FUNCTION_BLOCK IDENTControl_MF
VAR_INPUT
	pADR_IN:								PVOID;					(* Pointer array input data *)
	cbSIZE_IN:								UDINT;					(* Size array input data *)
	pADR_OUT:								PVOID;					(* Pointer array output data *)
	cbSIZE_OUT:								UDINT;					(* Size array output data *)
    I_T_Timeout 							: TIME := T#10S;   		// Timeout to check command responses
    I_b_StartRead 							: BOOL;   				// Trigger to start read command
    I_b_StartWrite 							: BOOL;   				// Trigger to start write command
    I_b_StartSpecialCommand 				: BOOL;   				// Trigger to start special command (user defined command)
    I_b_UserMemory_UID 						: BOOL;   				//0 := access to User Memory; 1 := access to UID/Fixcode
    I_b_EPC									: BOOL;					//0 := configuration done by Head1UserMemoryUID active; 1 := access to UII/EPC Code (UHF only)
	I_b_SingleEnhanced 						: BOOL;   				// 0 = Single command (one-time) ; 1 = Enhanced command (permanent)
    I_b_Quit 								: BOOL;   				// Trigger to start Quit command (abort Enhanced command)
    I_w_StartAddress 						: WORD;   				// Startaddress of memory access 
    I_i_WordNumber 							: INT;   				// Number of blocks
    I_w_TagType 							: WORD;    				// TagType
END_VAR
VAR_OUTPUT
	O_b_Done 								: BOOL;   				//0 = tag leave detection zone (Enhanced); 1 = tag access successfully executed
    O_b_NoDataCarrier 						: BOOL;   				//0 = tag inside/enter detection zone; 1 = no tag or tag leave detection zone
    O_b_Busy 								: BOOL;   				//0 = no command actiive; 1 = command active
    O_b_Finish 								: BOOL;   				//0 = command active; 1 = command finished
    O_b_Error 								: BOOL;   				//0 = no error state; 1 = error state active; check status value
    O_B_Status 								: BYTE;   				//Status value of the command response; error information
	O_B_ReplyCounter 						: BYTE;					//Counter of the command responses; increment each new response
END_VAR
   VAR_IN_OUT 
    IO_b_SetRestart 						: BOOL;   				//Trigger initialisation routine
    IO_b_InitFinish 						: BOOL;   				//Initialisation routine finished
	IO_b_NewData							: BOOL;  	
	UserData 								: IDENTControl_UserData_IUH_MF;//Data block for read/write data
 	END_VAR
VAR
	INDATA 									: ARRAY[0..253] OF BYTE;
	OUTDATA 								: ARRAY[0..253] OF BYTE;
	UpdateSlave_IN							: BOOL;
    MASK_UPDATEBIT_SLAVE 					: BYTE := 1;
    MASK_UPDATEBIT_MASTER 					: BYTE := 2;
    MASK_DELETEBIT 							: BYTE := 4;
	
	statEdgeA								: BOOL;
	statEdgeB								: BOOL;
	statFlagC								: BOOL;
	
	Counter_FP								: INT;
	
	Head_ExistTC							: BOOL;
	Head_NotExist							: BOOL;
	Head_Done								: BOOL;
	Head_Error								: BOOL;
	Head_Busy								: BOOL;
	Head_SglCmdActive						: BOOL;
	Head_EnhCmdActive						: BOOL;
	Head_QuitCmdActive						: BOOL;
	Head_ReadCmdActive						: BOOL;
	Head_SpecialCmdActive					: BOOL;
	Head_NewData							: BOOL;
	Head_TimeoutActive						: BOOL;
	Head_TimeoutOccurred					: BOOL;
	Head_TransfToHead						: BOOL;
	Head_SendOK								: BOOL;
	Head_Execute							: BOOL;
	Head_Receive_OK							: BOOL;
	Head_WriteCmdActive						: BOOL;
	
	RTRIG_Read:									R_TRIG;					(* function block detects positive edge Read Command *)
	RTRIG_Write: 								R_TRIG;					(* function block detects positive edge Write Command *)
	RTRIG_Quit : 								R_TRIG;					(* function block detects positive edge Quit Command *)
	RTRIG_SpecialCommand: 						R_TRIG;					(* function block detects positive edge Special Command *)
	RTRIG_SetRestart: 							R_TRIG;					(* function block detects positive edge SetRestart *)
	
	STATE_INIT 								: USINT;
    STATE_CMD 								: USINT;
	
	Watchdog:									TON;
	i										: INT := 0;
	FragmentCounter_1						: INT;
	StartReadDataTransmission				: Bool;
	SingleCommandFinished					: BOOL;
	NumberTags								: DWORD;
END_VAR

	(*
	#############################################################################################
	
	General Header
	------------------------------------------------------------------------------------------
	Short description:  Function Block for IC-KP2-2HB21-2V1D EtherCAT with MultiFrame Protocol
	Version:            3.0
	Name:               Function block for IC-KP2-2HB21-2V1D EtherCAT with MultiFrame Protocol
	Date:               2024-09-19
	Company:            Pepperl+Fuchs SE
	Author:             Karsten Reinhardt
	EMail:              kreinhardt@de.pepperl-fuchs.com
	Phone:              +49 (0) 621 776 1736
	
		Changes 3.0: first release
	    - based on the SingleFrame version with adoption to MultiFrame
		- contains further commands which not supported by the UHF system
		- reading and writing is done with the 16 Bit commands
	
	
	*)


(*Read in process data; copy into #INDATA structure*)
MEMCPY(ADR(INDATA), pADR_IN, cbSIZE_IN); (* Receive complete Input-Telegram from IdentControl *)

(* Check every cycle if a new telegram is available *)
	IF (((INDATA[0]) AND MASK_UPDATEBIT_SLAVE) = ((OUTDATA[0] AND MASK_UPDATEBIT_SLAVE))) THEN
	    Head_Receive_OK                                 := TRUE;    (* inform PLC, that a new telegram is available *)
	    
	ELSE
	    Head_Receive_OK                                 := FALSE;   (* inform PLC, that no new telegram is available *)
	END_IF;
	(*Copy Update slave bit into internal variable*)
	UpdateSlave_IN 										:= InData[0].0;
	(*Trigger for positive edge on Update slave bit*)
	statEdgeA 											:= UpdateSlave_IN AND NOT statFlagC;
	(*Trigger for negative edge on Update slave bit*)
	statEdgeB 											:= NOT UpdateSlave_IN AND statFlagC;
	
	statFlagC 											:= UpdateSlave_IN;
	
	//generate Testcounter
	IF (statEdgeA = TRUE) OR (statEdgeB = TRUE) THEN
	    Counter_FP 										:= Counter_FP + 1;     // increment each new response telegram
	END_IF;

	//--------------------------------------------
	
	       O_B_Status 							:= INDATA[4];
			O_B_ReplyCounter 					:= INDATA[5];	
	
		//first response telegram after send command
	    IF Counter_FP = 1 THEN
	        FragmentCounter_1 							:= 16#0;                  //Fragment counter of first response telegram                    
	        IF ((INDATA[4] = 16#00) OR (INDATA[4] = 16#04)) AND (INDATA[2] <> 16#02) THEN              //Status
	        FOR i:=0 TO 245 BY 1 DO
			UserData.ReadData[i]						:= INDATA[i+8];
			END_FOR;
				StartReadDataTransmission 				:= TRUE;
	        END_IF;
	        
	        IF FragmentCounter_1 >= 16#00 AND INDATA[4] = 16#00 THEN
	            O_b_NoDataCarrier 						:= FALSE;
	            O_b_Error 								:= FALSE;
	        END_IF;
	        
	        IF FragmentCounter_1 = 16#00 THEN
	            IF INDATA[4] = 16#05 THEN  // No Tag
	                HEAD_Done 							:= FALSE;
	                HEAD_NewData 						:= TRUE;
	                HEAD_Execute 						:= FALSE;
	                HEAD_TimeoutActive 					:= FALSE;
	                O_b_NoDataCarrier 					:= TRUE;
	                Counter_FP 							:= 16#00;
	             	//   O_B_Status 							:= INDATA[4];
					//	O_B_ReplyCounter 					:= INDATA[5];
	                O_b_Done 							:= FALSE;
	                O_b_Error 							:= FALSE;
					FOR i:=0 TO 55 BY 1 DO
					UserData.EPC_LeaveTag[i]			:= INDATA[i+8];
					END_FOR;
					IO_b_NewData 						:= TRUE;
	              //  IF #statEdge1 = True THEN
	            END_IF;
	            IF  INDATA[4] = 16#00 THEN
	                HEAD_Done 							:= FALSE;
	                HEAD_NewData 						:= TRUE;
	                HEAD_Execute 						:= FALSE;
	                HEAD_TimeoutActive 					:= FALSE;
	                O_b_NoDataCarrier 					:= FALSE;
	             //   O_B_Status 							:= INDATA[4];
				//	O_B_ReplyCounter 					:= INDATA[5];
	                O_b_Done 							:= TRUE;
	                O_b_Error 							:= FALSE;
					IO_b_NewData 						:= TRUE;
	              //  IF #statEdge1 = True AND #Resp_Telegram_1[5] <> 16#04 AND #Resp_Telegram_1[6] = 16#00  AND NOT #HEAD.QuitCmdActive = True THEN
	            END_IF;
	            IF  INDATA[4] = 16#0B THEN
					FOR i:=0 TO 4 BY 1 DO
					UserData.TagInformation[i]				:= INDATA[i+8];
					END_FOR;
					IO_b_NewData 						:= TRUE;
	            END_IF;
				IF HEAD_SglCmdActive = TRUE AND INDATA[4] = 16#0F  THEN
	                O_b_Finish 							:= TRUE;
	                O_b_Done 							:= TRUE;
	                O_b_Busy 							:= FALSE;
	                HEAD_SglCmdActive 					:= FALSE;
	                HEAD_ReadCmdActive 					:= FALSE;
					HEAD_WriteCmdActive 					:= FALSE;
					HEAD_TimeoutActive 					:= FALSE;
					HEAD_Busy 							:= FALSE;
					HEAD_Execute 						:= FALSE;
					FOR i:=0 TO 3 BY 1 DO
					UserData.NumberTags[i]				:= INDATA[i+8];
					END_FOR;
					NumberTags							:= SHL (BYTE_TO_DWORD(UserData.NumberTags[0]), 24) OR 
														SHL (BYTE_TO_DWORD(UserData.NumberTags[1]), 16) OR 
														SHL (BYTE_TO_DWORD(UserData.NumberTags[2]), 8) OR 
														BYTE_TO_DWORD(UserData.NumberTags[3]);
					IF Numbertags = 16#30303030 THEN
					O_b_NoDataCarrier 					:= TRUE;
	                Counter_FP 							:= 16#00;
	            //    O_B_Status 							:= INDATA[4];
				//	O_B_ReplyCounter 					:= INDATA[5];
	                O_b_Error 							:= FALSE;	
					END_IF;		
					IO_b_NewData 						:= TRUE;						
	            END_IF;
				IF HEAD_SglCmdActive = TRUE AND INDATA[4] = 16#04 THEN
	                O_b_Finish 							:= TRUE;
	                O_b_Done 							:= TRUE;
	                O_b_Busy 							:= FALSE;
	                HEAD_SglCmdActive 					:= FALSE;
	                HEAD_ReadCmdActive 					:= FALSE;
	                HEAD_TimeoutActive 					:= FALSE;
	                HEAD_Execute 						:= FALSE;
	                HEAD_Busy 							:= FALSE;
	                O_b_Error 							:= TRUE;
	            //    O_B_Status 							:= INDATA[4];
				//	O_B_ReplyCounter 					:= INDATA[5];
	           		IO_b_NewData 						:= TRUE;
				END_IF;
	            IF HEAD_EnhCmdActive = TRUE AND INDATA[4] = 16#04 THEN
	                O_b_Done 							:= TRUE;
	                HEAD_ReadCmdActive 					:= FALSE;
	                HEAD_TimeoutActive 					:= FALSE;
	                O_b_Error 							:= TRUE;
	             //   O_B_Status 							:= INDATA[4];
				//	O_B_ReplyCounter 					:= INDATA[5];
	                Counter_FP 							:= 16#00;
					IO_b_NewData 						:= TRUE;
	            END_IF;
				IF HEAD_WriteCmdActive = TRUE AND INDATA[4] = 16#00 THEN
					FOR i:=0 TO 55 BY 1 DO
					UserData.EPC_WrittenTag[i]			:= INDATA[i+8];
					END_FOR;
				END_IF;
				IF INDATA[4] = 16#04 THEN
					O_b_Error 							:= TRUE;
				//	O_B_Status 							:= INDATA[4];
				//	O_B_ReplyCounter 					:= INDATA[5];
				END_IF
	        END_IF;
	    END_IF;
		Counter_FP 										:= 16#00;
	
	//-------------------------------------------	
		
	
	(* PLC always copy the inverted Update Slave bit from INPUT to OUTPUT *)
	(*  is now allowed to send a new telegram *)
	OUTDATA[0]                                         	:= ((OutData[0] AND (NOT MASK_UPDATEBIT_SLAVE)) OR ((NOT InData[0]) AND MASK_UPDATEBIT_SLAVE));
	
	(* Define Trigger inputs as rising edges *)        
	RTRIG_SetRestart(CLK                               	:=  IO_b_SetRestart);      (*SetRestart Input*)
	RTRIG_Quit(CLK                                     	:=  I_b_Quit);             (*Quit Input*)
	RTRIG_Read(CLK                                     	:=  I_b_StartRead);        (*Read Input*)
	RTRIG_Write(CLK                                    	:=  I_b_StartWrite);       (*Write Input*)
	RTRIG_SpecialCommand(CLK                           	:=  I_b_StartSpecialCommand);   (*SpecialCommand Input*)
	
	
	(* Handling of the SetRestart Routine
	- routine consist of the flip of the Delete Bit and the execution of the Change Tag command
	*) 
	IF RTRIG_SetRestart.Q THEN                                                     (*Check positive edge on SetRestart input*)
	    STATE_INIT                                     	:= 1;
	    STATE_CMD                                      	:= 0;
	    Counter_FP                                     	:= 0;
	END_IF;
	
	CASE STATE_INIT OF
	        
	    0:  (* ********************** Idle state ******************* *)
	        ;
	    1:  (* ********************** Initialize variables  ******************* *)
	        
	        (*Reset internal variables and Outputs*) 
	        IO_b_InitFinish                            	:= FALSE;
	        HEAD_ExistTC                               	:= FALSE;
	        HEAD_NotExist                              	:= FALSE;
	        HEAD_Done                                  	:= FALSE;
	        O_b_Done                                   	:= FALSE;
	        HEAD_Error                                 	:= FALSE;
	        O_b_Error                                  	:= FALSE;
	        HEAD_Busy                                  	:= FALSE;
	        O_b_Busy                                   	:= FALSE;
	        HEAD_SglCmdActive                          	:= FALSE;
	        HEAD_EnhCmdActive                          	:= FALSE;
	        HEAD_QuitCmdActive                         	:= FALSE;
	        HEAD_ReadCmdActive                         	:= FALSE;
	        HEAD_SpecialCmdActive                      	:= FALSE;
	        HEAD_NewData                               	:= FALSE;
	        HEAD_TimeoutActive                         	:= FALSE;
	        HEAD_TimeoutOccurred                       	:= FALSE;
	        HEAD_TransfToHead                          	:= FALSE;
	        HEAD_SendOK                                	:= FALSE;
	        HEAD_Execute                               	:= FALSE;
	        HEAD_Receive_OK                            	:= FALSE;
	        HEAD_WriteCmdActive                        	:= FALSE;
	        O_b_NoDataCarrier                          	:= FALSE;
	        O_b_Finish                                 	:= FALSE;
			IO_b_NewData 									:= FALSE;
			
			FOR i:=0 TO 245 BY 1 DO
		    UserData.WriteData[i]                       := 16#00;
			END_FOR;
			FOR i:=0 TO 245 BY 1 DO
		    UserData.ReadData[i]                       := 16#00;
			END_FOR;
	        FOR i:=0 TO 3 BY 1 DO
		    UserData.NumberTags[i]                       := 16#00;
			END_FOR;
			FOR i:=0 TO 4 BY 1 DO
		    UserData.TagInformation[i]                       := 16#00;
			END_FOR;
			FOR i:=0 TO 55 BY 1 DO
		    UserData.EPC_WrittenTag[i]                       := 16#00;
			END_FOR;
			FOR i:=0 TO 55 BY 1 DO
		    UserData.EPC_LeaveTag[i]                       := 16#00;
			END_FOR;
	       
	        STATE_INIT                                 	:= STATE_INIT + 1;                 (* Go to next state *)
	        
	        Counter_FP := 0;
	
	        
	    2: (* ****************** Delete internal FIFO Memory / telegrams of IC-KP2-2HB21 *************** *)
	        
	        (* Set Deletebit *)
	        OutData[0]                                 	:= ((OutData[0] AND (NOT MASK_DELETEBIT)) OR ((NOT OutData[0]) AND MASK_DELETEBIT));    (* Delete old telegrams in identsystem *)
	        
	        STATE_INIT                                 	:= STATE_INIT + 1;                 (* Go to next state *)
	        
	    3: (* ******************** Wait for delete bit in INPUTS equals OUTPUTS **************** *)
	        
	        IF ((OutData[0] AND MASK_DELETEBIT) = (( InData[0] AND MASK_DELETEBIT))) THEN       (*Check if the value of the Delete Bit is identically in input and output*)
	            STATE_INIT                             	:= STATE_INIT + 1;                 (* Go to next state *)
	        END_IF;
	        
	    4: (* ***************** Send Change Tag Command; stop command execution *************** *)
	        
	        (* Configure Change Tag command in OutData structure *)
	        OutData[1]                                 	:= 16#00;           (*unused*)
	        OutData[2]                                 	:= 16#04;           (*CommandCode CT*)
	        OutData[3]                                 	:= 16#00;           (*unused*)
	        OutData[4]                                 	:= WORD_TO_BYTE(SHR(I_w_TagType,8));           (*TagType High Byte*)
	        OutData[5]                                 	:= WORD_TO_BYTE(I_w_TagType);           (*TagType Low Byte*)
			FOR i:=6 TO 253 BY 1 DO
		    OutData[i]                                 	:= 16#00;
			END_FOR;	        	        
	        HEAD_Busy                                  	:= TRUE;
	        O_b_Busy                                   	:= TRUE;
	        HEAD_Done                                  	:= FALSE;
	        O_b_Done                                   	:= FALSE;
	        HEAD_TimeoutActive                         	:= TRUE;
	        HEAD_SglCmdActive                          	:= TRUE;
	        HEAD_EnhCmdActive                          	:= FALSE;
	        HEAD_Execute                               	:= TRUE;
	        HEAD_TransfToHead                          	:= TRUE;
	        
	        (* Handling of Handshake process for sending a new command *)
	        (* Check if IC-KP2-2HB21 is able to receive a new telegram; 
	        IC-KP2-2HB21 is able to receive new telegrams if the value of the UpdateBit_Master of the Input and Output is different *)
	        IF ((OutData[0] AND MASK_UPDATEBIT_MASTER) <> (InData[0] AND MASK_UPDATEBIT_MASTER)) THEN  (* Receiver (IC-KP2-2HB21) accepts a new Telegram *)
	                        (* Invert Updatebit master in order to signalize a new telegram is available *)
	            OutData[0]                             	:= (OutData[0] AND (NOT MASK_UPDATEBIT_MASTER)) OR (InData[0] AND MASK_UPDATEBIT_MASTER);
	            HEAD_SendOK                            	:= TRUE;
	        ELSE
	            HEAD_SendOK                            	:= FALSE;  (* Receiver (IC-KP2-2HB21) doesnt't accept a new Telegram *)
	        END_IF;
	        
	        (* Send OutData field with Quit command to IC-KP2-2HB21 *)
	        IF HEAD_SendOK THEN
	            
	            HEAD_TransfToHead                      	:= FALSE;
	            STATE_INIT                             	:= STATE_INIT + 1; (* Go to next state *)
	        END_IF;
	        
	    5: (* ******************** Wait for Quit command response ************************ *)
	        IF HEAD_Receive_OK THEN (*If new telegram from IC-KP2-2HB21 is available*)
	            
	            HEAD_NewData                           	:= TRUE;
	           // O_B_Status                             	:= InData[4];          (*Copy received status value to Output variable Status*)
	           // O_B_ReplyCounter 					   	:= INDATA[5];
	            IF InData[4] = 16#0 THEN
	                HEAD_ExistTC                       	:= TRUE;
	                HEAD_NotExist                      	:= FALSE;
	            ELSE    (* Error *)
	                HEAD_ExistTC                       	:= FALSE;
	                HEAD_NotExist                      	:= FALSE;
	                HEAD_Error                         	:= TRUE;
	                O_b_Error                          	:= TRUE;
	            END_IF;
	            HEAD_Busy                              	:= FALSE;
	            O_b_Busy                               	:= FALSE;
	            HEAD_Done                              	:= TRUE;
	            O_b_Done                               	:= TRUE;
	            O_b_Finish                             	:= TRUE;
	            HEAD_SglCmdActive                      	:= FALSE;
	            HEAD_TimeoutActive                     	:= FALSE;
	            HEAD_Execute                           	:= FALSE;
	            STATE_INIT                             	:= STATE_INIT + 1; (* Go to next state *)
	        END_IF;
	        
	    6: (* Initialization finished  *)
	        IF HEAD_ExistTC (*OR #HEAD.NotExist*) THEN
	            IO_b_InitFinish                        	:= TRUE;
	            IO_b_SetRestart                        	:= FALSE;
	            STATE_INIT                             	:= 0; (* Go to idle state *)
	        END_IF;
	END_CASE;
		
	
(*  ******************************************************************** Command Processing [Communication routine]   ****************************************************************************************************   *)
	IF IO_b_InitFinish THEN
	    
	    (* ********** Commands ********** *)
	    IF NOT HEAD_Execute THEN
	        
	        IF RTRIG_Quit.Q OR RTRIG_Read.Q OR RTRIG_Write.Q OR RTRIG_SpecialCommand.Q THEN
	            (* Discard previous #RECORD_DATA.INPUT content, except CONTROL Byte *)
	            FragmentCounter_1                      	:= 16#00;
	            SingleCommandFinished                  	:= FALSE;
	            O_b_NoDataCarrier                      	:= FALSE;
	            //Reset Error output with trigger on new command
	            HEAD_Error                             	:= FALSE;
	            O_b_Error                              	:= FALSE;
	            								
	              (* ***** Quit ***** *)
	            IF RTRIG_Quit.Q THEN
					OutData[1]                         	:= 16#00;           (*unused*)
	        		OutData[2]                         	:= 16#02;           (*CommandCode Quit QU*)
	        		OutData[3]                         	:= 16#00;           (*unused*)
	        		OutData[4]                         	:= 16#00;           (*unused*)
	        		OutData[5]                         	:= 16#00;           (*unused*)
	        		OutData[6]                         	:= 16#00;           (*unused*)
	        		OutData[7]                         	:= 16#00;           (*unused*)
					FOR i:=8 TO 253 BY 1 DO
		    		OutData[i]                         	:= 16#00;
					END_FOR;
	               (* HEAD_QuitCmdActive 					:= TRUE;
	                HEAD_EnhCmdActive 					:= FALSE;
	                HEAD_TransfToHead 					:= TRUE;
	                STATE_CMD 							:= 1;*)
				HEAD_QuitCmdActive                     := TRUE;
	            HEAD_SpecialCmdActive                  := FALSE;
	            HEAD_EnhCmdActive                      := FALSE;
	            HEAD_TransfToHead                      := TRUE;
	            HEAD_WriteCmdActive                    := FALSE;
	            HEAD_ReadCmdActive                     := FALSE;
	            STATE_CMD                              := 1;
	            END_IF;
	            				
	              (* ***** Special Command ***** *)
	            IF RTRIG_SpecialCommand.Q THEN
	                FOR i:=2 TO 32 BY 1 DO
		    		OutData[i]                        	:= UserData.SpecialCommand[i-2];
					END_FOR;
					//MOVE_BLK(IN := #UserData.SpecialCommand[0],  OUT => #OutData[1],  COUNT := 31);
	                HEAD_SpecialCmdActive              	:= TRUE;
	                HEAD_EnhCmdActive                  	:= FALSE;
	                HEAD_WriteCmdActive                	:= FALSE;
	                HEAD_ReadCmdActive                 	:= FALSE;
	                HEAD_TransfToHead                  	:= TRUE;
	                STATE_CMD                          	:= 1;
	            END_IF;
	            
	            (* ***** Single Read 2-Byte Words ***** *)
	            IF RTRIG_Read.Q = TRUE AND I_b_UserMemory_UID = FALSE (*AND #I_b_EPC = False*) AND I_b_SingleEnhanced = FALSE THEN
					OutData[1]                        	:= 16#00;           (*unused*)
	        		OutData[2]                        	:= 16#49;           (*CommandCode Single Read 2-Byte Words #SR*)
	        		OutData[3]                         	:= 16#00;           (*unused*)
	        		OutData[4]                        	:= WORD_TO_BYTE(SHR(I_w_StartAddress,8));        (*StartAddress High Byte*)
	        		OutData[5]                        	:= WORD_TO_BYTE(I_w_StartAddress);           	(*StartAddress Low Byte*)
	        		OutData[6]                        	:= INT_TO_BYTE(SHR(I_i_WordNumber,8));           (*WordNumber High Byte*)
	        		OutData[7]                        	:= INT_TO_BYTE(I_i_WordNumber); 					(*WordNumber Low Byte*)
					FOR i:=8 TO 253 BY 1 DO
		    		OutData[i]                         	:= 16#00;
					END_FOR;	                
                    HEAD_SglCmdActive                  	:= TRUE;
	                HEAD_EnhCmdActive                  	:= FALSE;
	                HEAD_WriteCmdActive                	:= FALSE;
	                HEAD_ReadCmdActive                 	:= TRUE;
	                HEAD_TransfToHead                  	:= TRUE;
	                STATE_CMD                          	:= 1;
	            END_IF;
	            				
	            (* **** Enhanced Read 2-Byte Words ***** *)
	            IF RTRIG_Read.Q = TRUE AND I_b_UserMemory_UID = FALSE (*AND #I_b_EPC = False*) AND I_b_SingleEnhanced = TRUE THEN
					OutData[1]                         	:= 16#00;           (*unused*)
	        		OutData[2]                         	:= 16#4B;           (*CommandCode Enhanced Read 2-Byte Words #ER*)
	        		OutData[3]                        	:= 16#00;           (*unused*)
	        		OutData[4]                        	:= WORD_TO_BYTE(SHR(I_w_StartAddress,8));        (*StartAddress High Byte*)
	        		OutData[5]                         	:= WORD_TO_BYTE(I_w_StartAddress);           	(*StartAddress Low Byte*)
	        		OutData[6]                        	:= INT_TO_BYTE(SHR(I_i_WordNumber,8));           (*WordNumber High Byte*)
	        		OutData[7]                        	:= INT_TO_BYTE(I_i_WordNumber); 					(*WordNumber Low Byte*)	
					FOR i:=8 TO 253 BY 1 DO
		    		OutData[i]                         	:= 16#00;
					END_FOR;                                               (*Overwrite unused part of field with 16#00*)
	                HEAD_SglCmdActive                  	:= FALSE;
	                HEAD_EnhCmdActive                  	:= TRUE;
	                HEAD_WriteCmdActive                	:= FALSE;
	                HEAD_ReadCmdActive                 	:= TRUE;
	                HEAD_TransfToHead                  	:= TRUE;
	                STATE_CMD                          	:= 1;
	            END_IF;
	            							
	            (* ***** Single Read Fixcode (UID/TID) ***** *)
	            IF RTRIG_Read.Q = TRUE AND I_b_UserMemory_UID = TRUE (*AND #I_b_EPC = False*) AND I_b_SingleEnhanced = FALSE THEN
					OutData[1]                        	:= 16#00;           (*unused*)
	        		OutData[2]                       	:= 16#01;           (*CommandCode Single Read Fixcode (UID/TID) SF*)
	        		OutData[3]                        	:= 16#00;           (*unused*)
	        		OutData[4]                        	:= 16#00;           (*unused*)
	        		OutData[5]                          := 16#00;           (*unused*)
	        		OutData[6]                         	:= 16#00;           (*unused*)
	        		OutData[7]                         	:= 16#00;           (*unused*)
					FOR i:=8 TO 253 BY 1 DO
		    		OutData[i]                         	:= 16#00;
					END_FOR;                                               (*Overwrite unused part of field with 16#00*)
	                HEAD_SglCmdActive                  	:= TRUE;
	                HEAD_EnhCmdActive                  	:= FALSE;
	                HEAD_WriteCmdActive                	:= FALSE;
	                HEAD_ReadCmdActive                 	:= TRUE;
	                HEAD_TransfToHead                  	:= TRUE;
	                STATE_CMD                          	:= 1;
	            END_IF;
	            								
	            (* ***** Enhanced Read Fixcode (UID/TID) ***** *)
	            IF RTRIG_Read.Q = TRUE AND I_b_UserMemory_UID = TRUE (*AND #I_b_EPC = False*) AND I_b_SingleEnhanced = TRUE THEN
					OutData[1]                        	:= 16#00;           (*unused*)
	        		OutData[2]                         	:= 16#1D;           (*CommandCode Enhanced Read Fixcode (UID/TID) EF*)
	        		OutData[3]                         	:= 16#00;           (*unused*)
	        		OutData[4]                      	:= 16#00;           (*unused*)
	        		OutData[5]                       	:= 16#00;           (*unused*)
	        		OutData[6]                        	:= 16#00;           (*unused*)
	        		OutData[7]                         	:= 16#00;           (*unused*)
					FOR i:=8 TO 253 BY 1 DO
		    		OutData[i]                         	:= 16#00;
					END_FOR;                                                (*Overwrite unused part of field with 16#00*)
	                HEAD_SglCmdActive                  	:= FALSE;
	                HEAD_EnhCmdActive                  	:= TRUE;
	                HEAD_WriteCmdActive                	:= FALSE;
	                HEAD_ReadCmdActive                 	:= TRUE;
	                HEAD_TransfToHead                  	:= TRUE;
	                STATE_CMD                          	:= 1;
	            END_IF;	           		

	            (* **** Single Read UII (EPC/UII) ***** *)
	            IF RTRIG_Read.Q = TRUE AND I_b_UserMemory_UID = FALSE AND I_b_EPC = TRUE AND I_b_SingleEnhanced = FALSE THEN
					OutData[1]                    		:= 16#00;           (*unused*)
	        		OutData[2]                         	:= 16#D2;           (*CommandCode Single Read UII (EPC/UII) SN*)
	        		OutData[3]                        	:= 16#00;           (*unused*)
	        		OutData[4]                        	:= 16#00;           (*unused*)
	        		OutData[5]                         	:= 16#00;           (*unused*)
	        		OutData[6]                        	:= 16#00;           (*unused*)
	        		OutData[7]                       	:= 16#00;           (*unused*)
					FOR i:=8 TO 253 BY 1 DO
		    		OutData[i]                         	:= 16#00;
					END_FOR;                                               (*Overwrite unused part of field with 16#00*)
	                HEAD_SglCmdActive                  	:= TRUE;
	                HEAD_EnhCmdActive                  	:= FALSE;
	                HEAD_WriteCmdActive                	:= FALSE;
	                HEAD_ReadCmdActive                 	:= TRUE;
	                HEAD_TransfToHead                  	:= TRUE;
	                STATE_CMD                          	:= 1;                         
	            END_IF;	            		

	            (* ***** Enhanced Read UII (EPC/UII) ***** *)
	            IF RTRIG_Read.Q = TRUE AND I_b_UserMemory_UID = FALSE AND I_b_EPC = TRUE AND I_b_SingleEnhanced = TRUE THEN
					OutData[1]                       	:= 16#00;           (*unused*)
	        		OutData[2]                       	:= 16#D3;           (*CommandCode Single Read UII (EPC/UII) SN*)
	        		OutData[3]                       	:= 16#00;           (*unused*)
	        		OutData[4]                        	:= 16#00;           (*unused*)
	        		OutData[5]                       	:= 16#00;           (*unused*)
	        		OutData[6]                        	:= 16#00;           (*unused*)
	        		OutData[7]                        	:= 16#00;           (*unused*)
					FOR i:=8 TO 253 BY 1 DO
		    		OutData[i]                         	:= 16#00;
					END_FOR;                                                  (*Overwrite unused part of field with 16#00*)
	                HEAD_SglCmdActive                  	:= FALSE;
	                HEAD_EnhCmdActive                  	:= TRUE;
	                HEAD_WriteCmdActive                	:= FALSE;
	                HEAD_ReadCmdActive                 	:= TRUE;
	                HEAD_TransfToHead                  	:= TRUE;
	                STATE_CMD                          	:= 1;
	            END_IF;	                      				
				
	            (* ***** Single Write 2-Byte Words ***** *)
	            IF RTRIG_Write.Q = TRUE AND I_b_UserMemory_UID = FALSE (*AND #I_b_EPC = False*) AND I_b_SingleEnhanced = FALSE THEN
					OutData[1]                        	:= 16#00;           (*unused*)
	        		OutData[2]                         	:= 16#4A;           (*CommandCode Single Write 2-Byte Words #SW*)
	        		OutData[3]                         	:= 16#00;           (*unused*)
	        		OutData[4]                         	:= WORD_TO_BYTE(SHR(I_w_StartAddress,8));        (*StartAddress High Byte*)
	        		OutData[5]                         	:= WORD_TO_BYTE(I_w_StartAddress);           	(*StartAddress Low Byte*)
	        		OutData[6]                         	:= INT_TO_BYTE(SHR(I_i_WordNumber,8));           (*WordNumber High Byte*)
	        		OutData[7]                         	:= INT_TO_BYTE(I_i_WordNumber); 					(*WordNumber Low Byte*)
					FOR i:=8 TO 253 BY 1 DO
		    		OutData[i]                         	:= UserData.WriteData[i-8];
					//OutData[i]                                 := WriteData[i-8];
					END_FOR;                               (*Copy WriteData field to output field*)
	                HEAD_SglCmdActive                  	:= TRUE;
	                HEAD_WriteCmdActive                	:= TRUE;
	                HEAD_ReadCmdActive                 	:= FALSE;
	                HEAD_EnhCmdActive                  	:= FALSE;
	                HEAD_TransfToHead                  	:= TRUE;
	                STATE_CMD                          	:= 1;
	            END_IF;	            
				
	            (* ***** Enhanced Write 2-Byte Words ***** *)
	            IF RTRIG_Write.Q = TRUE AND I_b_UserMemory_UID = FALSE (*AND #I_b_EPC = False*) AND I_b_SingleEnhanced = TRUE THEN
					OutData[1]                       	:= 16#00;           (*unused*)
	        		OutData[2]                         	:= 16#4C;           (*CommandCode Enhanced Write Word EW*)
	        		OutData[3]                         	:= 16#00;           (*unused*)
	        		OutData[4]                         	:= WORD_TO_BYTE(SHR(I_w_StartAddress,8));        (*StartAddress High Byte*)
	        		OutData[5]                         	:= WORD_TO_BYTE(I_w_StartAddress);           	(*StartAddress Low Byte*)
	        		OutData[6]                         	:= INT_TO_BYTE(SHR(I_i_WordNumber,8));           (*WordNumber High Byte*)
	        		OutData[7]                          := INT_TO_BYTE(I_i_WordNumber); 					(*WordNumber Low Byte*)
					FOR i:=8 TO 253 BY 1 DO
		    		OutData[i]                          := UserData.WriteData[i-8];
					//OutData[i]                                 := WriteData[i-8];
					END_FOR;                               (*Copy WriteData field to output field*)                            (*Copy WriteData field to output field*)
	                HEAD_SglCmdActive                  	:= FALSE;
	                HEAD_WriteCmdActive                	:= TRUE;
	                HEAD_ReadCmdActive                 	:= FALSE;
	                HEAD_EnhCmdActive                  	:= TRUE;
	                HEAD_TransfToHead                  	:= TRUE;
	                STATE_CMD                          	:= 1;
	            END_IF;
	            
				(* ***** Single Write Fixcode ***** *)
	            IF RTRIG_Write.Q = TRUE AND I_b_UserMemory_UID = TRUE (*AND #I_b_EPC = False*) AND I_b_SingleEnhanced = FALSE THEN
					OutData[1]                          := 16#00;           (*unused*)
	        		OutData[2]                          := 16#1F;           (*CommandCode Single Write Fixcode SX*)
	        		OutData[3]                          := 16#00;           (*unused*)
	        		OutData[4]                          := 16#31; //WORD_TO_BYTE(SHR(I_w_StartAddress,8));        (*StartAddress High Byte*)
	        		OutData[5]                          := 16#31; //WORD_TO_BYTE(I_w_StartAddress);           	(*StartAddress Low Byte*)
	        		OutData[6]                          := 16#0; //INT_TO_BYTE(SHR(I_i_WordNumber,8));           (*WordNumber High Byte*)
	        		OutData[7]                          := 16#5; //INT_TO_BYTE(I_i_WordNumber); 					(*WordNumber Low Byte*)
					FOR i:=8 TO 253 BY 1 DO
		    		OutData[i]                          := UserData.WriteData[i-8];
					//OutData[i]                                 := WriteData[i-8];
					END_FOR;                               (*Copy WriteData field to output field*)
	                HEAD_SglCmdActive                  	:= TRUE;
	                HEAD_WriteCmdActive                	:= TRUE;
	                HEAD_ReadCmdActive                 	:= FALSE;
	                HEAD_EnhCmdActive                  	:= FALSE;
	                HEAD_TransfToHead                  	:= TRUE;
	                STATE_CMD                          	:= 1;
	            END_IF;
								
	            (* ***** Enhanced Write Fixcode ***** *)
	            IF RTRIG_Write.Q = TRUE AND I_b_UserMemory_UID = TRUE (*AND #I_b_EPC = False*) AND I_b_SingleEnhanced = TRUE THEN
					OutData[1]                      	:= 16#00;           (*unused*)
	        		OutData[2]                        	:= 16#24;           (*CommandCode Enhanced Write Word EW*)
	        		OutData[3]                          := 16#00;           (*unused*)
	        		OutData[4]                          := 16#31; //WORD_TO_BYTE(SHR(I_w_StartAddress,8));        (*StartAddress High Byte*)
	        		OutData[5]                          := 16#31; //WORD_TO_BYTE(I_w_StartAddress);           	(*StartAddress Low Byte*)
	        		OutData[6]                          := 16#0; //INT_TO_BYTE(SHR(I_i_WordNumber,8));           (*WordNumber High Byte*)
	        		OutData[7]                          := 16#5; //INT_TO_BYTE(I_i_WordNumber); 					(*WordNumber Low Byte*)
					FOR i:=8 TO 253 BY 1 DO
		    		OutData[i]                          := UserData.WriteData[i-8];
					//OutData[i]                                 := WriteData[i-8];
					END_FOR;                               (*Copy WriteData field to output field*)                            (*Copy WriteData field to output field*)
	                HEAD_SglCmdActive                  	:= FALSE;
	                HEAD_WriteCmdActive                	:= TRUE;
	                HEAD_ReadCmdActive                 	:= FALSE;
	                HEAD_EnhCmdActive                  	:= TRUE;
	                HEAD_TransfToHead                  	:= TRUE;
	                STATE_CMD                          	:= 1;
	            END_IF;				
				
				(* ***** Single Program Special Fixcode ***** *)
	            IF RTRIG_Write.Q = TRUE AND I_b_UserMemory_UID = FALSE AND I_b_EPC = TRUE AND I_b_SingleEnhanced = FALSE THEN
					OutData[1]                    		:= 16#00;           (*unused*)
	        		OutData[2]                        	:= 16#0D;           (*CommandCode Single Program Special Fixcode*)
	        		OutData[3]                          := 16#00;           (*unused*)
	        		OutData[4]                        	:= 16#00; //WORD_TO_BYTE(SHR(I_w_StartAddress,8));        (*StartAddress High Byte*)
	        		OutData[5]                          := 16#00; //WORD_TO_BYTE(I_w_StartAddress);           	(*StartAddress Low Byte*)
	        		OutData[6]                          := INT_TO_BYTE(SHR(I_i_WordNumber,8));           (*WordNumber High Byte*)
	        		OutData[7]                          := INT_TO_BYTE(I_i_WordNumber); 						(*WordNumber Low Byte*)			
					FOR i:=8 TO 63 BY 1 DO
		    		OutData[i]                                 := UserData.WriteData[i-8];
					END_FOR;                              (*Copy WriteData field to output field*)
	                HEAD_SglCmdActive                  := TRUE;
	                HEAD_WriteCmdActive                := TRUE;
	                HEAD_ReadCmdActive                 := FALSE;
	                HEAD_EnhCmdActive                  := FALSE;
	                HEAD_TransfToHead                  := TRUE;
	                STATE_CMD                          := 1;
	            END_IF;
				
				IF  RTRIG_Read.Q OR RTRIG_Write.Q OR RTRIG_SpecialCommand.Q THEN
					FOR i:=0 TO 245 BY 1 DO
					UserData.ReadData[i]				:= 16#00;
					END_FOR;
				
				
				
				
				
				(*
	            (*
	            (* **** Single Write EPC/UII ***** *)
	            IF #RTRIG_Write.Q = True AND #I_b_UserMemory_TID = False AND #I_b_EPC = True AND #I_b_SingleEnhanced = FALSE THEN
	                #OutData[1]                         := INT_TO_BYTE(#I_i_ByteNumber) + 16#07;                            (*Frame Length*)
	                #OutData[2]                         := 16#00;                                                           (*Fragmentation Counter*)
	                #OutData[3]                         := 16#00;                                                           (*Telegram Length High byte*)
	                #OutData[4]                         := INT_TO_BYTE(#I_i_ByteNumber) + 16#04;                            (*Telegram Length Low Byte*)
	                #OutData[5]                         := 16#CE;                                                           (* Command: Single Write EPC/UII*)
	                #OutData[6]                         := INT_TO_BYTE(#I_i_ByteNumber);                                    (*Length of EPC Information; 2 Byte PC Word + EPC/UII*)
	                MOVE_BLK(IN := #UserData.WriteData[0], OUT => #OutData[7],  COUNT := 22);                              (*Copy WriteData field to output field*)
	                #HEAD.SglCmdActive                  := TRUE;
	                #HEAD.WriteCmdActive                := True;
	                #HEAD.ReadCmdActive                 := FALSE;
	                #HEAD.EnhCmdActive                  := FALSE;
	                #HEAD.TransfToHead                  := TRUE;
	                #STATE_CMD                          := 1;
	            END_IF;
	            *)
	            
	        END_IF;
	        
	        IF #RTRIG_Quit.Q THEN
	            //Reset Error if Quit command triggered
	            #HEAD.Error                             := FALSE;
	            #O_b_Error                              := False;
	            
	              (* ***** Quit ***** *)
	            #OutData[1]                             := 16#06;                                                           (*Frame Length*)
	            #OutData[2]                             := 16#00;                                                           (*Fragmentation Counter*)
	            #OutData[3]                             := 16#00;                                                           (*Telegram Length High byte*)
	            #OutData[4]                             := 16#03;                                                           (*Telegram Length Low Byte*)
	            #OutData[5]                             := 16#02;                                                           (* Command: QUIT *)
	            FILL_BLK(IN := 16#0, COUNT := 28,  OUT => #OutData[6]);
	            #HEAD.QuitCmdActive                     := True;
	            #HEAD.SpecialCmdActive                  := FALSE;
	            #HEAD.EnhCmdActive                      := FALSE;
	            #HEAD.TransfToHead                      := TRUE;
	            #HEAD.WriteCmdActive                    := FALSE;
	            #HEAD.ReadCmdActive                     := FALSE;
	            #STATE_CMD                              := 1;*)
	        
				END_IF;
			END_IF; 
	    END_IF;


	    
	            (* ***** Handle communication and analysis ***** *)
	            CASE STATE_CMD OF
	                    
	                0: (* ***** Idle state ***** *)
	                    ;
	                1:(* ***** Execution ***** *)
	                    IF HEAD_TransfToHead THEN
	                        HEAD_Busy                  := TRUE;
	                        O_b_Busy                   := TRUE;
	                        HEAD_Done                  := FALSE;
	                        O_b_Done                   := FALSE;
	                        O_b_Finish                 := FALSE;
	                        HEAD_SendOK                := FALSE;
	                        HEAD_Receive_OK             := FALSE;
	                        HEAD_NewData               := FALSE;
	                        HEAD_TimeoutActive         := TRUE;
	                        HEAD_TimeoutOccurred       := FALSE;
	                        HEAD_Execute               := TRUE;
	                        O_b_NoDataCarrier          := FALSE;
	                        O_b_Finish                 := FALSE;
	                        
	                        (* ***** Handshake-WRITE ***** *)
	                        (* Check if IC-KP2-2HB21 is able to receive a new telegram *)
	                        IF ((OutData[0] AND MASK_UPDATEBIT_MASTER) <> (InData[0] AND MASK_UPDATEBIT_MASTER)) THEN
	                            (* Receiver (IC-KP2-2HB21) accepts a new Telegram *)
	                            
	                            (* Invert Updatebit master in order to signalize a new telegram is available *)
	                            OutData[0]             := (OutData[0] AND (NOT MASK_UPDATEBIT_MASTER)) OR (InData[0] AND MASK_UPDATEBIT_MASTER);
	                            HEAD_SendOK            := TRUE;
	                            
	                            //Test KReinhardt 2023-06-28
	                            Counter_FP             := 0;
	                           
	                        ELSE
	                            (* Receiver (IC-KP2-2HB21) doesnt't accept a new Telegram *)
	                            HEAD_SendOK            := FALSE;
	                        END_IF;
	                        
	                            (* Send CMD to identsystem *)
	                        IF HEAD_SendOK THEN
	
	                            HEAD_TransfToHead      := FALSE;
	                            STATE_CMD              := STATE_CMD + 1; (* Go to next state *)
	                        END_IF;
	                    END_IF;
	                    
	                    
	                2:(* ***** Analyze InData ***** *)
	                    (* Receive Telegram *)
	                    IF HEAD_Receive_OK THEN //(ReceiveTelegram(ChannelLocal := nChannel) = TRUE ) THEN
	                        HEAD_NewData               := TRUE;
	                        
	                        (* Data carrier detected *)
	                        IF InData[4] = 16#0  OR InData[4] = 16#B THEN
	                            HEAD_Done              := TRUE;
	                        (* No data carrier detected *)
	                       // ELSIF #InData[6] = 16#5 THEN
	                       //     #O_b_NoDataCarrier      := TRUE;
	                       //     #HEAD.Done              := False;
	                        END_IF;
	                        
	                        //Status 16#00 response during Quit command or Special command -> command successfully finished
	                        IF InData[4] = 16#0 AND HEAD_QuitCmdActive = TRUE THEN
	                            HEAD_Done              := TRUE;
	                            O_b_Done               := TRUE;
	                            O_b_Finish             := TRUE;
	                            HEAD_Busy              := FALSE;
	                            O_b_Busy               := FALSE;
	                            HEAD_NewData           := FALSE;
	                            HEAD_QuitCmdActive     := FALSE;
	                            HEAD_Execute           := FALSE;
	                            HEAD_TimeoutActive     := FALSE;
	                            STATE_CMD              := 0; (* Go to idle state *)
	                            O_b_NoDataCarrier      := FALSE;
	                            O_b_Finish             := TRUE;
								IO_b_NewData 		   := TRUE;
	                        END_IF;
	                        
	                        //Status 16#00 response during  Special command -> command successfully finished
	                        IF InData[4] = 16#0 AND HEAD_SpecialCmdActive = TRUE THEN
	                            HEAD_Done              := TRUE;
	                            O_b_Done               := TRUE;
	                            HEAD_Busy              := FALSE;
	                            O_b_Busy               := FALSE;
	                            HEAD_NewData           := FALSE;
	                            HEAD_SpecialCmdActive  := FALSE;
	                            HEAD_Execute           := FALSE;
	                            HEAD_TimeoutActive     := FALSE;
	                            STATE_CMD              := 0; (* Go to idle state *)
	                            O_b_NoDataCarrier      := FALSE;
	                            O_b_Finish             := TRUE;
								IO_b_NewData 		   := TRUE;
	                        END_IF;
	                        
	                        IF InData[4] = 16#F AND HEAD_SpecialCmdActive = TRUE THEN
	                            HEAD_Done := TRUE;
	                            O_b_Done := TRUE;
	                            HEAD_Busy := FALSE;
	                            O_b_Busy := FALSE;
	                            HEAD_NewData := FALSE;
	                            HEAD_SpecialCmdActive := FALSE;
	                            HEAD_Execute := FALSE;
	                            HEAD_TimeoutActive := FALSE;
	                            STATE_CMD := 0; (* Go to idle state *)
	                            O_b_NoDataCarrier := TRUE;
	                            O_b_Finish := TRUE;
								IO_b_NewData 		   := TRUE;
	                        END_IF;
	                        
	                        //Status 16#04 response during Quit command or Special command -> Error
	                        IF InData[4] = 16#4 AND HEAD_QuitCmdActive = TRUE OR HEAD_SpecialCmdActive = TRUE THEN
	                            HEAD_Done              := TRUE;
	                            O_b_Done               := TRUE;
	                            HEAD_Busy              := FALSE;
	                            O_b_Busy               := FALSE;
	                            HEAD_NewData           := FALSE;
	                            HEAD_QuitCmdActive     := FALSE;
	                            HEAD_Execute           := FALSE;
	                            HEAD_TimeoutActive     := FALSE;
	                            STATE_CMD              := 0; (* Go to idle state *)
	                            O_b_NoDataCarrier      := FALSE;
	                            O_b_Finish             := TRUE;
								HEAD_SpecialCmdActive  := FALSE;					
	                        END_IF;
	                        
	  
	                        //Status 16#00 response during write command -> contains EPC information of written tag
	                        IF InData[4] = 16#0 AND HEAD_WriteCmdActive = TRUE THEN
	                            STATE_CMD              := 2; (* Go to idle state *)
	                         //   MOVE_BLK(IN := #InData[7], OUT => #UserData.UID_WrittenTag[0], COUNT := 25);
	                        END_IF;
	                    END_IF;
	            END_CASE;
	        END_IF;

	
	
	(* ***** Watchdog ***** *)
		
Watchdog(IN:=Head_TimeoutActive, PT:= I_T_Timeout);

	        IF WATCHDOG.Q THEN
	            HEAD_TimeoutActive                     := FALSE;
	            HEAD_TimeoutOccurred                   := TRUE;
	            HEAD_SendOK                            := FALSE;
	            HEAD_Receive_OK                         := FALSE;
	            HEAD_SglCmdActive                      := FALSE;
	            HEAD_EnhCmdActive                      := FALSE;
	            HEAD_Execute                           := FALSE;
	            HEAD_TransfToHead                      := FALSE;
	            HEAD_Error                             := TRUE;
	            O_b_Error                              := TRUE;
	            HEAD_Busy                              := FALSE;
	            O_b_Busy                               := FALSE;
	            HEAD_Done                              := TRUE;
	            O_b_Done                               := TRUE;
	        END_IF;

			MEMCPY(pADR_OUT, ADR(OUTDATA[0]), cbSIZE_OUT);

END_FUNCTION_BLOCK
